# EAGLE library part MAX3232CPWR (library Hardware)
RS-232 Line Driver/Receiver
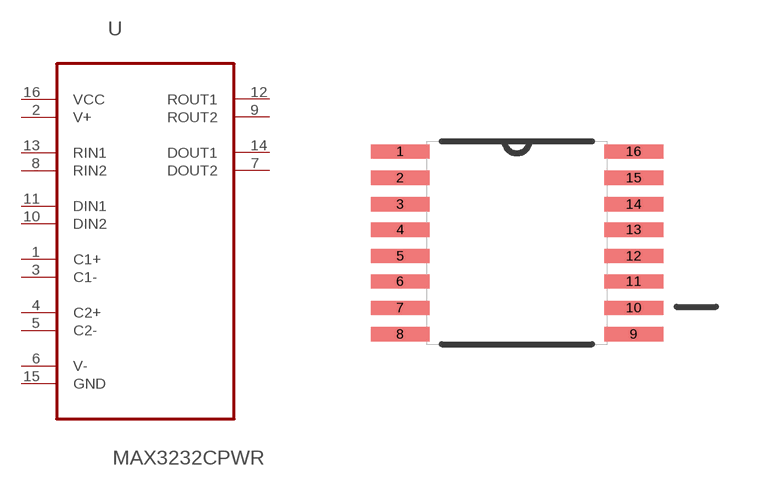
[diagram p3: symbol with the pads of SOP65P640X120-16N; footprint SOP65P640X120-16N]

Designator prefix U

## MAX3232CPWR (MPN: MAX3232CPWR; OC_FARNELL: 1460372; OC_NEWARK: 75C1004; PACKAGE: TSSOP-16; SUPPLIER: Texas Instruments)  [SOP65P640X120-16N]
1  C1+  pas
2  V+  pwr
3  C1-  pas
4  C2+  pas
5  C2-  pas
6  V-  pwr
7  DOUT2  out
8  RIN2  in
9  ROUT2  out
10  DIN2  in
11  DIN1  in
12  ROUT1  out
13  RIN1  in
14  DOUT1  out
15  GND  pas
16  VCC  pwr

## Footprint SOP65P640X120-16N (pad centres in mm)
smd 1.473 x 0.356: 1 -2.921,2.286; 2 -2.921,1.626; 3 -2.921,0.965; 4 -2.921,0.33; 5 -2.921,-0.33; 6 -2.921,-0.965; 7 -2.921,-1.626; 8 -2.921,-2.286; 9 2.921,-2.286; 10 2.921,-1.626; 11 2.921,-0.965; 12 2.921,-0.33; 13 2.921,0.33; 14 2.921,0.965; 15 2.921,1.626; 16 2.921,2.286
